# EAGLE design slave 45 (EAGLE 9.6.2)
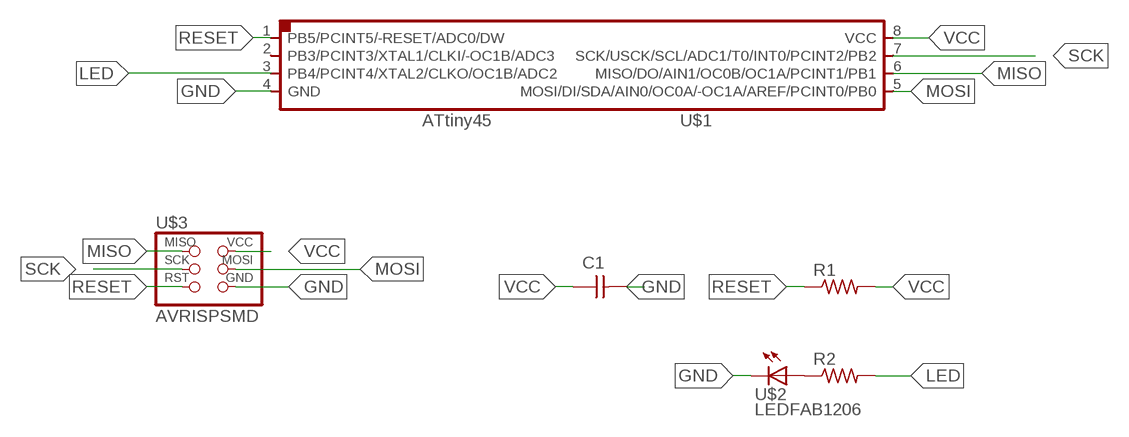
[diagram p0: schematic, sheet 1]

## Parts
C1  CAP-UNPOLARIZEDFAB  [C1206FAB]
R1  RES-US1206FAB  [R1206FAB]
R2  RES-US1206FAB  [R1206FAB]
U$1  ATTINY45SI  [SOIC8]
U$2  LEDFAB1206  [LED1206FAB]
U$3  AVRISPSMD  [2X03SMD]

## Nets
GND: C1.2 U$1.4(GND) U$2.2(C) U$3.6(GND)
LED: R2.2 U$1.3(PB4/PCINT4/XTAL2/CLKO/OC1B/ADC2)
MISO: U$1.6(MISO/DO/AIN1/OC0B/OC1A/PCINT1/PB1) U$3.1(MISO)
MOSI: U$1.5(MOSI/DI/SDA/AIN0/OC0A/-OC1A/AREF/PCINT0/PB0) U$3.4(MOSI)
N$1: R2.1 U$2.1(A)
RESET: R1.1 U$1.1(PB5/PCINT5/-RESET/ADC0/DW) U$3.5(RST)
SCK: U$1.7(SCK/USCK/SCL/ADC1/T0/INT0/PCINT2/PB2) U$3.3(SCK)
VCC: C1.1 R1.2 U$1.8(VCC) U$3.2(VCC)
Unconnected: U$1.2(PB3/PCINT3/XTAL1/CLKI/-OC1B/ADC3)

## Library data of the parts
C1 = fab:CAP-UNPOLARIZED
R1 R2 = fab:RES-US: Resistor (US Symbol)
U$1 = fab:ATTINY45
U$2 = fab:LED: LED
U$3 = fab:AVRISP

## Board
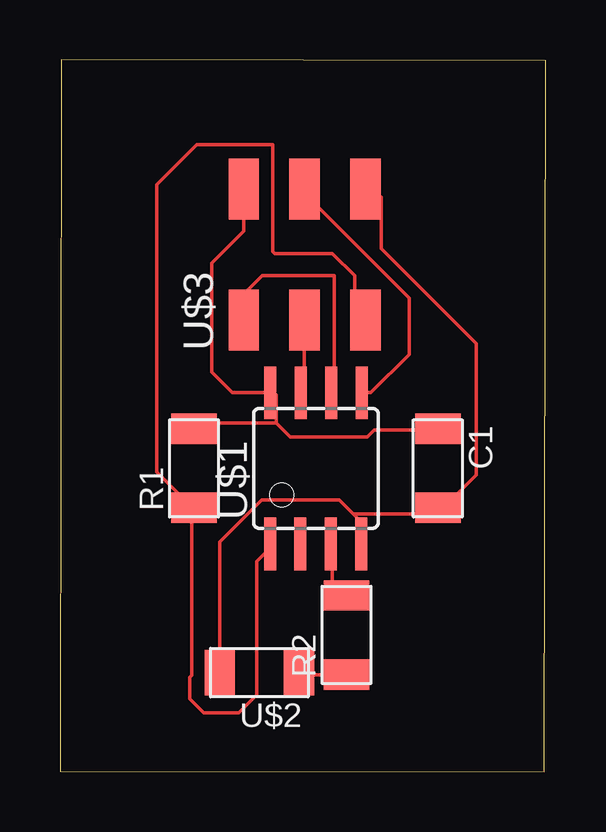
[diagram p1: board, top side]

Size 20.25 x 29.69 mm. Coordinates in mm from the lower left corner, seen from the top.
Outline: 0,0.03 20.19,0 20.25,29.66 0.06,29.69 0,0.03
Copper layers (1*16): Top 0.035mm / dielectric 1.5mm / Bottom 0.035mm
Design rules "default *": minimum track width 6mil, minimum drill 0.35mm, track to track 17mil, track to pad 17mil, pad to pad 6mil, via to via 6mil, smd to smd 6mil, copper to edge 40mil, drill to drill 6mil, minimum pad ring 10mil, minimum via ring 8mil, stop-mask expansion 4mil, vias tented up to drill 0mil, thermal gap 10mil

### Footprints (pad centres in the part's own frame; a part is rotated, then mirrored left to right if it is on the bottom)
C1206FAB = smd 1.27 x 1.905: 1 -1.651,0; 2 1.651,0
R1206FAB = smd 1.27 x 1.905: 1 -1.651,0; 2 1.651,0
SOIC8 = smd 0.5 x 2.2: 1 -1.905,-3.154; 2 -0.645,-3.154; 3 0.625,-3.154; 4 1.895,-3.154; 5 1.905,3.154; 6 0.635,3.154; 7 -0.635,3.154; 8 -1.905,3.154
LED1206FAB = smd 1.27 x 1.905: 1 -1.651,0; 2 1.651,0
2X03SMD = smd 2.54 x 1.27: 1 -2.54,2.54; 2 2.92,2.54; 3 -2.54,0; 4 2.92,0; 5 -2.54,-2.54; 6 2.92,-2.54

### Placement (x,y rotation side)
C1  15.74,12.66 270 top
R1  5.58,12.66 90 top
R2  11.93,5.71 90 top
U$1  10.66,12.66 0 top
U$2  8.31,4.15 180 top
U$3  10.2,21.38 90 top

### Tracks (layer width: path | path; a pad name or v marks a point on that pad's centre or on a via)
GND
  Top 0.152: 12.21,10.76 12.51,10.46 12.51,9.59 U$1.4 | 12.21,10.76 11.63,11.34 8.42,11.34 6.66,9.59 U$2.2 | 12.21,10.76 15.72,10.76 C1.2 16.01,11.05 17.34,12.38 17.34,17.87 13.38,21.83 13.38,23.98 U$3.6
LED
  Top 0.152: R2.2 11.64,7.36 11.34,7.67 11.34,9.3 U$1.3
MISO
  Top 0.152: U$1.6 11.43,16.51 11.43,20.7 8.43,20.7 7.66,19.93 U$3.1
MOSI
  Top 0.152: U$1.5 12.96,15.81 14.55,17.41 14.55,19.76 10.2,24.12 U$3.4
N$1
  Top 0.152: R2.1 10.04,4.06 9.96,3.98 U$2.1
RESET
  Top 0.152: U$1.1 8.71,9.3 8.19,8.78 8.19,3.21 7.45,2.47 5.99,2.47 5.41,3.06 5.41,3.95 5.5,4.04 5.5,10.76 R1.1 5.5,11.05 4.04,12.51 4.04,24.48 5.71,26.16 8.86,26.16 8.86,21.7 8.95,21.61 11.35,21.61 12.27,20.69 12.27,19.3 U$3.5
SCK
  Top 0.152: U$1.7 10.17,16.01 10.17,18.81 U$3.3
VCC
  Top 0.152: 9,14.55 9.59,13.97 12.8,13.97 13.09,14.26 15.72,14.26 C1.1 | 9,14.55 9,15.72 U$1.8 7.18,15.81 6.33,16.67 6.33,21.22 7.66,22.56 U$3.2 | 9,14.55 5.79,14.55 R1.2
